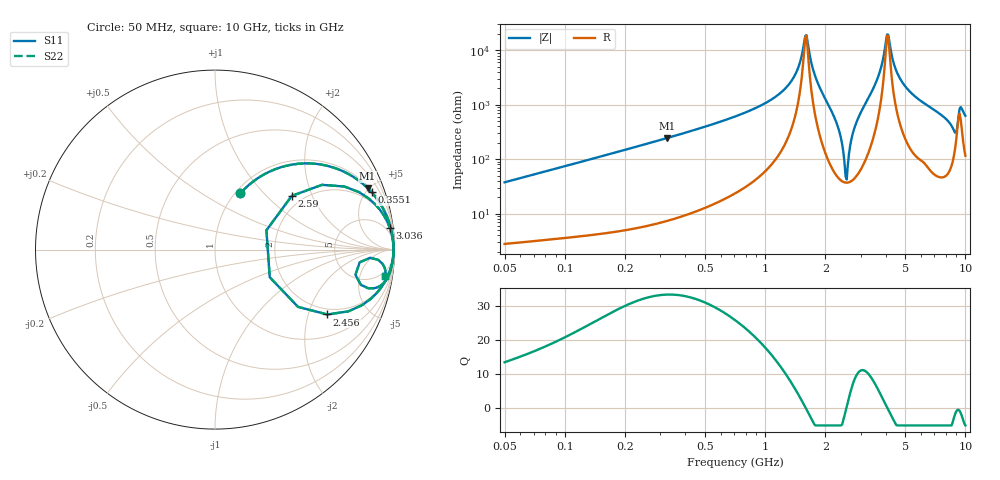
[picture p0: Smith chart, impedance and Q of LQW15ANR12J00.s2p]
!Murata Part Number: LQW15ANR12J00
!These Parameters are Measured in Series Mode Connection
!  o--[Z]--o
!Port1  Port2
!  o-------o
!Freq. Start=50[MHz] Stop=10[GHz], 401[Steps]
# Hz S RI R 50
!Freq.(Hz)	S 11(Real)	S 11(Imag)	S 21(Real)	S 21(Imag)	S 12(Real)	S 12(Imag)	S 22(Real)	S 22(Imag)
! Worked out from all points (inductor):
!   401 points, 50 MHz to 10 GHz, reference 50 ohm
!   read as one part in series: L = 119 nH near 51.34 MHz
!   highest Q = 33.4 at 323.7 MHz (marker M1), where L = 120 nH
!   self-resonance near 1.586 GHz
!   S11 on the Smith chart (normalised r, x): 50 MHz: 1.06, +0.75; 355.1 MHz: 1.16, +5.40; 2.456 GHz: 1.77, -2.67; 2.59 GHz: 1.74, +1.43; 3.036 GHz: 2, +16; 10 GHz: 3, -12
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5e7  0.1414 0.3134  0.8586 -0.3134  0.8586 -0.3134  0.1414 0.3134
1.214486e8  0.4508 0.4767  0.5492 -0.4767  0.5492 -0.4767  0.4508 0.4767
2.949953e8  0.8242 0.3659  0.1758 -0.3659  0.1758 -0.3659  0.8242 0.3659
3.236556e8  0.8498 0.3426  0.1502 -0.3426  0.1502 -0.3426  0.8498 0.3426
3.551004e8  0.8724 0.319  0.1276 -0.319  0.1276 -0.319  0.8724 0.319
7.071068e8  0.9679 0.158  0.0321 -0.158  0.0321 -0.158  0.9679 0.158
1.26648e9  0.9928 0.0484  0.00719 -0.0484  0.00719 -0.0484  0.9928 0.0484
1.445853e9  0.9947 0.0224  0.00534 -0.0224  0.00534 -0.0224  0.9947 0.0224
1.586325e9  0.995 0.00195  0.00502 -0.00195  0.00502 -0.00195  0.995 0.00195
1.717543e9  0.9943 -0.0186  0.00574 0.0186  0.00574 0.0186  0.9943 -0.0186
2.268358e9  0.9381 -0.1932  0.0619 0.1932  0.0619 0.1932  0.9381 -0.1932
2.455993e9  0.6257 -0.3614  0.3743 0.3614  0.3743 0.3614  0.6257 -0.3614
2.589628e9  0.4277 0.2992  0.5723 -0.2992  0.5723 -0.2992  0.4277 0.2992
2.766943e9  0.8923 0.2526  0.1077 -0.2526  0.1077 -0.2526  0.8923 0.2526
3.035766e9  0.9734 0.1225  0.0266 -0.1225  0.0266 -0.1225  0.9734 0.1225
4.062795e9  0.9951 0.00147  0.00485 -0.00147  0.00485 -0.00147  0.9951 0.00147
4.171863e9  0.9952 -0.00493  0.00481 0.00493  0.00481 0.00493  0.9952 -0.00493
4.577181e9  0.9946 -0.0258  0.00539 0.0258  0.00539 0.0258  0.9946 -0.0258
5.437278e9  0.9907 -0.0624  0.00934 0.0624  0.00934 0.0624  0.9907 -0.0624
8.759398e9  0.8553 -0.2159  0.1447 0.2159  0.1447 0.2159  0.8553 -0.2159
9.48396e9  0.933 -0.0786  0.067 0.0786  0.067 0.0786  0.933 -0.0786
1e10  0.9495 -0.1443  0.0505 0.1443  0.0505 0.1443  0.9495 -0.1443
